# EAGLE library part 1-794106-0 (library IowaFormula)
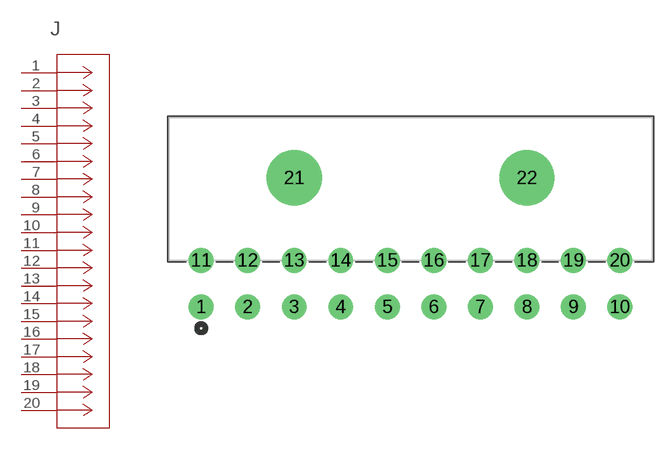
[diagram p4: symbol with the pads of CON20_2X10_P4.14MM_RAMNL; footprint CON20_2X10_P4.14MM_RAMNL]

Designator prefix J

## 1-794106-0 (MANUFACTURER_PART_NUMBER: 17941060; VENDOR: TE Connectivity)  [CON20_2X10_P4.14MM_RAMNL]
1  1  pas
2  2  pas
3  3  pas
4  4  pas
5  5  pas
6  6  pas
7  7  pas
8  8  pas
9  9  pas
10  10  pas
11  11  pas
12  12  pas
13  13  pas
14  14  pas
15  15  pas
16  16  pas
17  17  pas
18  18  pas
19  19  pas
20  20  pas

## Footprint CON20_2X10_P4.14MM_RAMNL (pad centres in mm)
drill 1.473 pad 1.981: 1 -37.262,-4.14; 2 -33.122,-4.14; 3 -28.981,-4.14; 4 -24.841,-4.14; 5 -20.701,-4.14; 6 -16.561,-4.14; 7 -12.421,-4.14; 8 -8.28,-4.14; 9 -4.14,-4.14; 10 0,-4.14; 11 -37.262,0; 12 -33.122,0; 13 -28.981,0; 14 -24.841,0; 15 -20.701,0; 16 -16.561,0; 17 -12.421,0; 18 -8.28,0; 19 -4.14,0; 20 0,0
drill 3.912 pad 3.912: 21 -28.981,7.341; 22 -8.28,7.341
